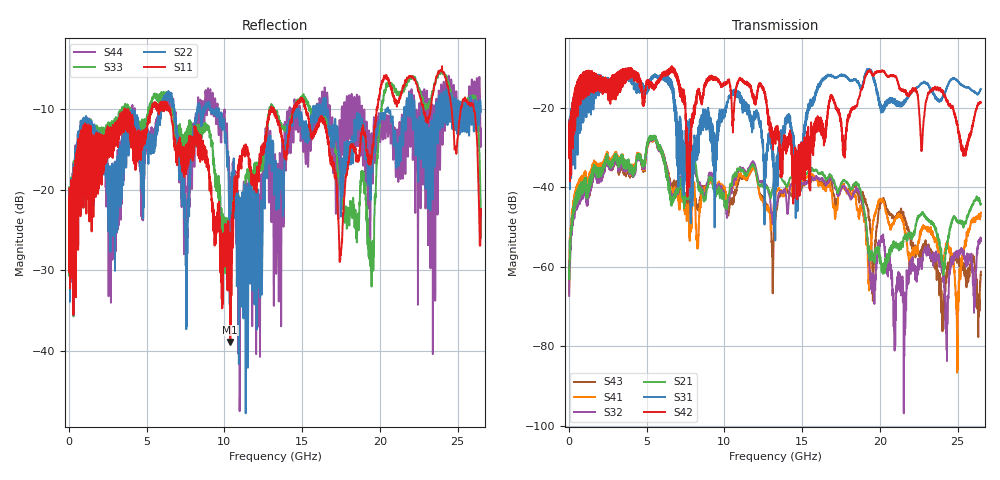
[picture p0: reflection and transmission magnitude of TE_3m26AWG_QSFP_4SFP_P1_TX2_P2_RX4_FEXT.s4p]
!Agilent Technologies,N5222A,MY51421691,A.10.00.00
!Agilent N5222A: A.10.00.00
!Date: Friday, January 30, 2015 12:38:12
!Correction: S11(Full 4 Port(1,2,3,4))
!S12(Full 4 Port(1,2,3,4))
!S13(Full 4 Port(1,2,3,4))
!S14(Full 4 Port(1,2,3,4))
!S21(Full 4 Port(1,2,3,4))
!S22(Full 4 Port(1,2,3,4))
!S23(Full 4 Port(1,2,3,4))
!S24(Full 4 Port(1,2,3,4))
!S31(Full 4 Port(1,2,3,4))
!S32(Full 4 Port(1,2,3,4))
!S33(Full 4 Port(1,2,3,4))
!S34(Full 4 Port(1,2,3,4))
!S41(Full 4 Port(1,2,3,4))
!S42(Full 4 Port(1,2,3,4))
!S43(Full 4 Port(1,2,3,4))
!S44(Full 4 Port(1,2,3,4))
!S4P File: Measurements: <S11,S12,S13,S14>,
!<S21,S22,S23,S24>,
!<S31,S32,S33,S34>,
!<S41,S42,S43,S44>:
# Hz S  dB  R 50.0
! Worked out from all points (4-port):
!   2650 points, 10 MHz to 26.5 GHz, reference 50 ohm
!   strongest paths, dB at 10 MHz, 6.63 GHz, 13.26 GHz, 19.88 GHz, 26.5 GHz:
!     S42: -25.0, -10.7, -25.1, -10.8, -18.7
!     S31: -24.7, -15.5, -42.4, -17.3, -15.3
!     S21: -60.5, -43.9, -38.1, -55.5, -44.2
!     S32: -67.3, -43.1, -45.4, -54.5, -53.3
!     S41: -66.7, -41.8, -42.8, -44.0, -46.4
!     S43: -64.9, -40.6, -48.5, -48.0, -61.2
!   lowest |S11| = -38.9 dB at 10.38 GHz (marker M1), VSWR 1.02, Z = 49.1 + j0.687 ohm
!   |S11| at or under -10 dB: start of sweep to 3.579 GHz; 6.486 GHz to 12.98 GHz (6.492 GHz wide, 66.7 % of centre); 15.24 GHz to 19.79 GHz (4.549 GHz wide, 26 % of centre)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
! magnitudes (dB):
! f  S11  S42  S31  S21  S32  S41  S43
! 10 MHz  -19.8  -25.0  -24.7  -60.5  -67.3  -66.7  -64.9
! 5.28 GHz  -10.3  -14.2  -12.3  -28.1  -28.1  -28.5  -28.4
! 10.38 GHz  -38.9  -14.4  -17.6  -39.1  -40.6  -40.2  -43.4
! 13.3 GHz  -11.1  -25.4  -36.2  -37.7  -45.0  -41.8  -47.1
! 16.61 GHz  -13.4  -22.0  -12.1  -37.7  -39.0  -39.7  -38.3
! 24.97 GHz  -14.3  -24.0  -13.2  -48.2  -56.2  -86.6  -58.1
! 26.5 GHz  -22.4  -18.7  -15.3  -44.2  -53.3  -46.4  -61.2
